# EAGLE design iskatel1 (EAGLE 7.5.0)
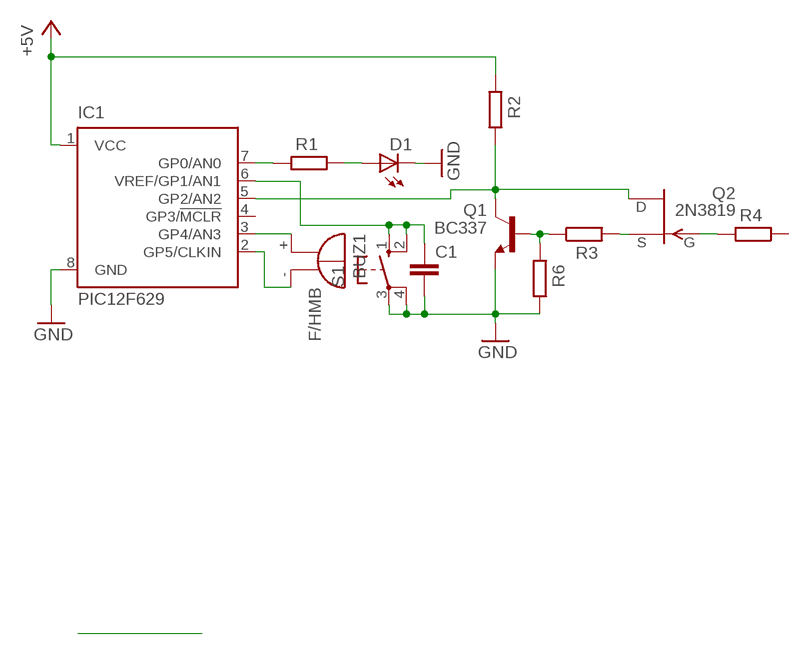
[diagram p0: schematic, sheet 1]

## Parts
BUZ1  F/HMB  [F/HMB]
C1  C-EUC1206  [C1206]
D1  LED5MM  [LED5MM]
IC1  PIC12F629  PIC12F675P  [DIL8]
Q1  BC337  [TO92]
Q2  2N3819  [TO92]
R1  R-EU_0204/7  [0204/7]
R2  R-EU_0207/10  [0207/10]
R3  R-EU_0204/7  [0204/7]
R4  R-EU_0204/7  [0204/7]
R6  R-EU_0204/7  [0204/7]
S1  10-XX  [B3F-10XX]

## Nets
+5V: IC1.1(VCC) R2.2
GND: C1.2 D1.K(C) IC1.8(GND) Q1.1(E) R6.1 S1.3(P) S1.4(P1)
N$1: BUZ1.+ IC1.3(GP4/AN3)
N$2: BUZ1.- IC1.2(GP5/CLKIN)
N$3: IC1.7(GP0/AN0) R1.2
N$4: D1.A R1.1
N$5: IC1.5(GP2/AN2) Q1.3(C) Q2.1(D) R2.1
N$6: Q1.2(B) R3.1 R6.2
N$8: Q2.3(S) R3.2
N$9: C1.1 IC1.6(VREF/GP1/AN1) S1.1(S) S1.2(S1)
N$10: Q2.2(G) R4.2
Unconnected: IC1.4(GP3/!MCLR) R4.1

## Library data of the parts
BUZ1 = buzzer:F/HMB: BUZZER; OC_FARNELL: unknown; OC_NEWARK: unknown
C1 = rcl:C-EU: CAPACITOR, European symbol
D1 = led:LED: LED
IC1 = microchip:PIC12F675: 8-Pin FLASH-Based 8-Bit CMOS Microcontroller Precision Internal 4 MHz oscillator factory calibrated to ±1% Low Power Features: Standby Current: - 1 nA @ 2.0V, typical Operating Current: - 8.5&micro;A @ 32 kHz, 2.0V, typical - 100&micro;A @ 1 MHz, 2.0V, typical Watchdog Timer Current: - 300 nA @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; MF: MICROCHIP; MPN: PIC12F675-E/P; OC_FARNELL: 9759018; OC_NEWARK: 92C4340
Q1 = transistor:BC337: NPN TRANSISTOR
Q2 = transistor-fet:2N3819: N-Channel Junction FET
R1-R4 R6 = rcl:R-EU_: RESISTOR, European symbol
S1 = switch-omron:10-XX: OMRON SWITCH; MPN: B3F-1000; OC_FARNELL: 176432; OC_NEWARK: 36M3542

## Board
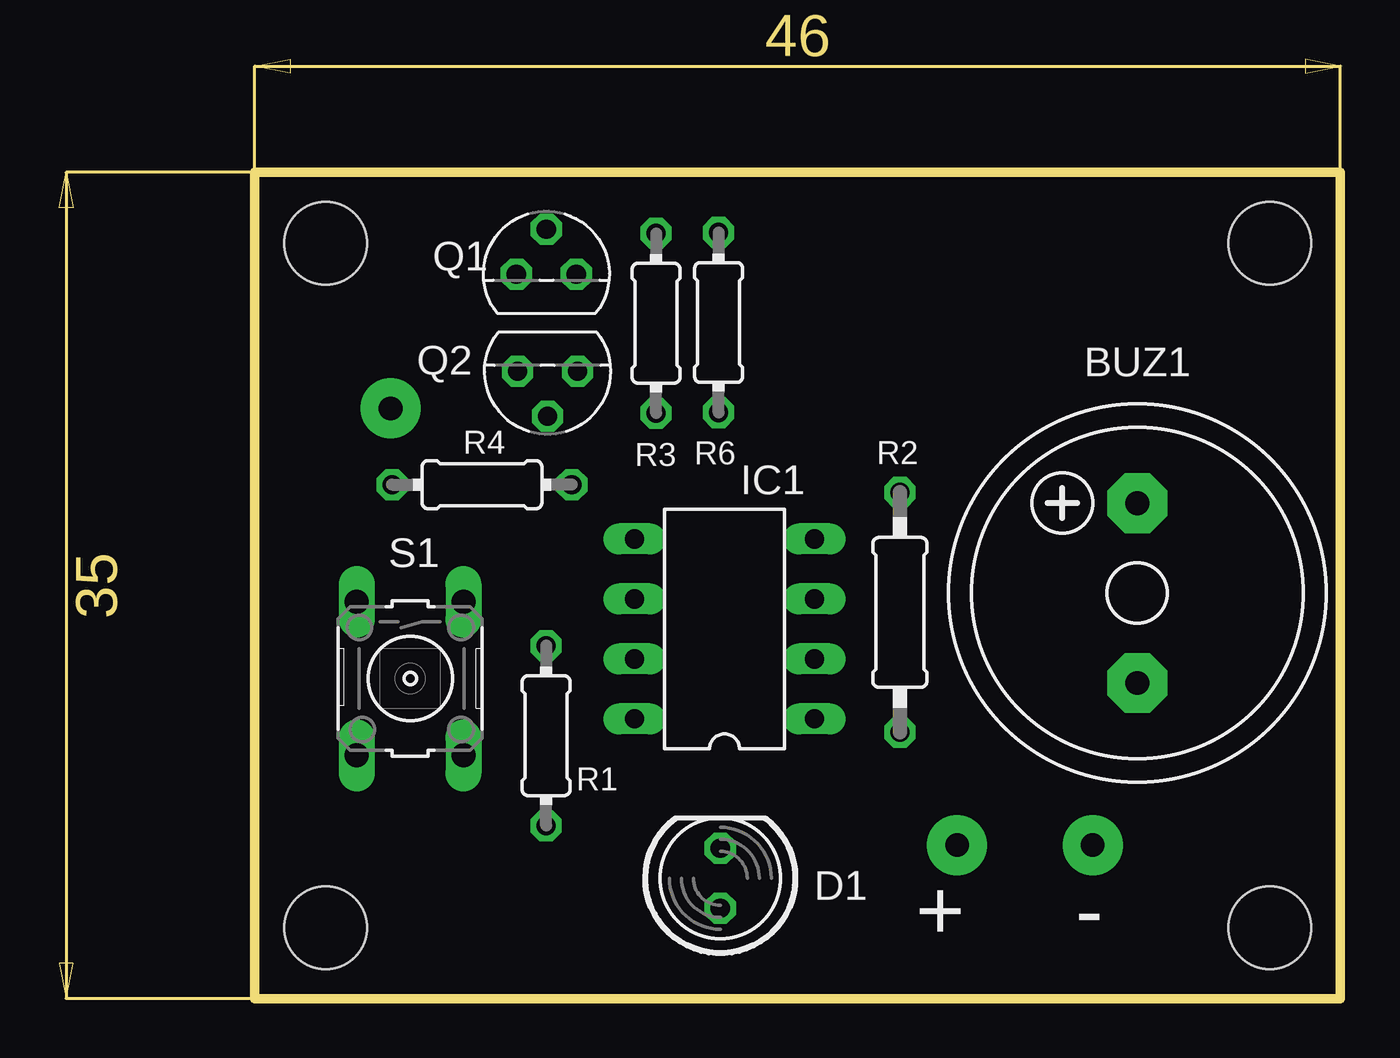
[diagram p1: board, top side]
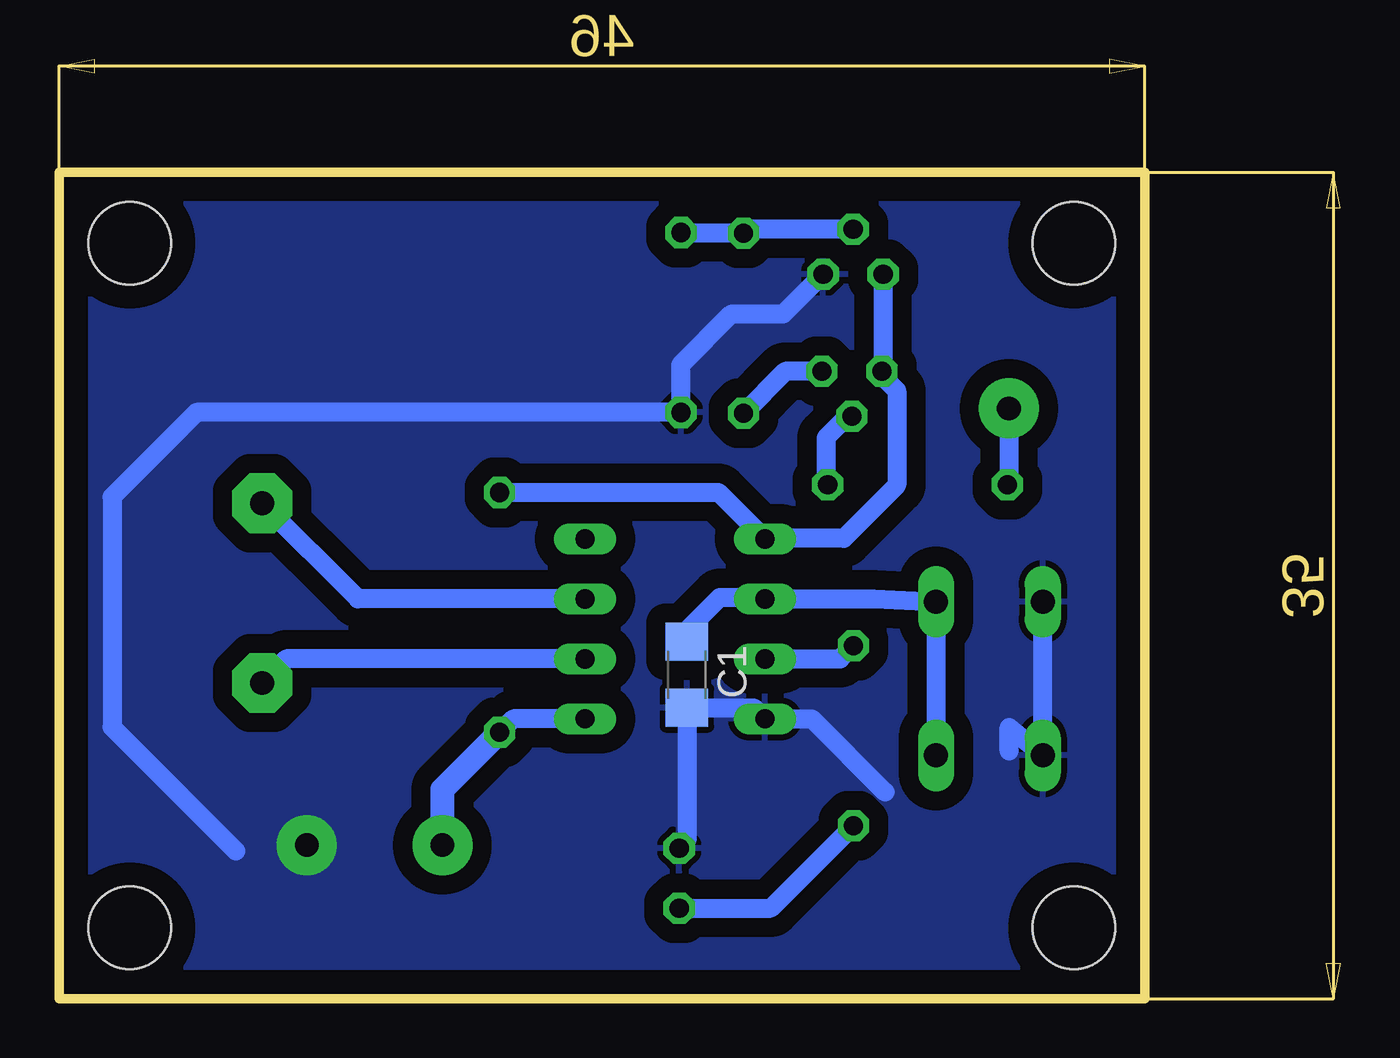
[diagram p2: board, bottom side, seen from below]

Size 54.3 x 39.8 mm. Coordinates in mm from the lower left corner, seen from the top.
Outline: 8.3,0 8.3,35 54.3,35 54.3,0 8.3,0
Copper layers (1*16): Top 0.035mm / dielectric 1.5mm / Bottom 0.035mm
Design rules "default": minimum track width 10mil, minimum drill 24mil, track to track 8mil, track to pad 8mil, pad to pad 8mil, via to via 8mil, smd to smd 8mil, copper to edge 40mil, drill to drill 8mil, minimum pad ring 10mil, minimum via ring 8mil, stop-mask expansion 4mil, vias tented up to drill 0mil, thermal gap 10mil
Holes 3.5 mm at 11.3,32 51.3,32 51.3,3 11.3,3

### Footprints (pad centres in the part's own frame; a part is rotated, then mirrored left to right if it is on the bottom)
F/HMB = drill 1.016 pad 2.54 octagon: + 3.81,0; - -3.81,0
C1206 = smd 1.6 x 1.8: 1 -1.4,0; 2 1.4,0
LED5MM = drill 0.813 octagon: A -1.27,0; K 1.27,0
DIL8 = drill 0.813 long: 1 -3.81,-3.81; 2 -1.27,-3.81; 3 1.27,-3.81; 4 3.81,-3.81; 5 3.81,3.81; 6 1.27,3.81; 7 -1.27,3.81; 8 -3.81,3.81
TO92 = drill 0.813 octagon: 1 1.27,0; 2 0,1.905; 3 -1.27,0
0204/7 = drill 0.813 octagon: 1 -3.81,0; 2 3.81,0
0207/10 = drill 0.813 octagon: 1 -5.08,0; 2 5.08,0
B3F-10XX = drill 1.016 long: 1 -3.251,2.261; 2 3.251,2.261; 3 -3.251,-2.261; 4 3.251,-2.261

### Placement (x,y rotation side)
BUZ1  45.69,17.18 90 top
C1  27.7,13.72 270 bottom
D1  28.02,5.1 90 top
IC1  28.2,15.66 90 top
Q1  20.65,30.69 0 top
Q2  20.7,26.57 180 top
R1  20.64,11.14 90 top
R2  35.63,16.36 270 top
R3  25.3,28.61 270 top
R4  17.92,21.77 0 top
R6  27.95,28.64 90 top
S1  14.88,13.56 270 top

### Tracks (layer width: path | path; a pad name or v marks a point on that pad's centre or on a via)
+5V  (via drill 1 pad 2.54)
  Bottom 0.813: IC1.1 35.06,11.85 R2.2
  Bottom 1.016: v38.05,6.5 38.05,8.86 R2.2
GND  (via drill 1 pad 2.54)
  Bottom 0.813: Q1.1 23.61,29 25.8,29 27.95,26.85 R6.1 48.47,24.83 52.05,21.25 52.05,11.5 46.8,6.25 | 19.3,8.75 22.4,11.85 IC1.8 24.86,12.32 C1.2 27.7,6.69 D1.K 28.14,6.25 | 14.05,10.5 14.05,11.49 S1.4 S1.3
  other vias: 43.8,6.5
  pour Bottom (isolate 0.813): 8.8,34.5 53.8,34.5 53.8,0.5 8.8,0.5
N$1
  Bottom 0.813: IC1.3 41.63,16.93 BUZ1.+
N$2
  Bottom 0.813: IC1.2 44.67,14.39 BUZ1.-
N$3
  Bottom 0.813: IC1.7 21.2,14.39 R1.2
N$4
  Bottom 0.813: D1.A 24.14,3.83 R1.1
N$5
  Bottom 0.813: R2.1 26.36,21.44 IC1.5 24.36,19.5 21.05,19.5 18.8,21.75 18.8,25.75 19.43,26.38 Q2.1 19.38,26.62 Q1.3
N$6
  Bottom 0.813: 20.51,32.45 Q1.2 25.12,32.59 R3.1 25.33,32.45 R6.2
N$8
  Bottom 0.813: Q2.3 23.53,26.57 R3.2
N$9
  Bottom 0.813: C1.1 27.7,15.6 26.3,17 24.46,17 IC1.6 19.77,16.93 S1.1 S1.2
N$10
  Bottom 0.813: Q2.2 20.89,24.66 21.8,23.75 21.8,21.84 R4.2
N$11  (via drill 1 pad 2.54)
  Bottom 0.813: v14.05,25 14.05,21.75

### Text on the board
tNames: + | -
